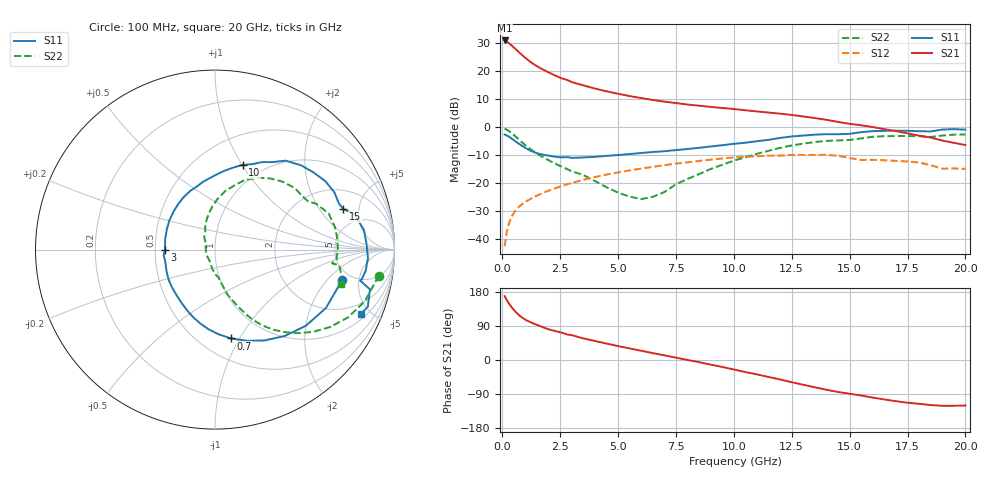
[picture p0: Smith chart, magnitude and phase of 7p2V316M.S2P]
! Infineon Technologies  Discrete & RF Semiconductors
! bfp620
! VCE =  2.3 V,  IC =  16 mA
! Common Emitter S-Parameters:  Sep 2002
# GHz  S  MA  R  50
!  f  S11  S21  S12  S22
! GHz  MAG  ANG  MAG  ANG  MAG  ANG  MAG  ANG
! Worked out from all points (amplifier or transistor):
!   59 points, 100 MHz to 20 GHz, reference 50 ohm
!   highest |S21| = 30.8 dB at 100 MHz (marker M1)
!   |S21| within 3 dB of that: start of sweep to 564.6 MHz
!   unconditionally stable (mu >= 1): 3.515 GHz to 10.17 GHz; 17.14 GHz to end of sweep
!   at 1 GHz: K = 0.65, MSG = 25.7 dB, |S12| = -26.8 dB
!   at 5.5 GHz: K = 1.05, MAG = 12.0 dB, |S12| = -15.6 dB
!   at 20 GHz: K = 1.27, MAG = 1.1 dB, |S12| = -15.0 dB
!   S11 on the Smith chart (normalised r, x): 100 MHz: 4.12, -2.98; 700 MHz: 0.70, -0.92; 3 GHz: 0.56, +0.00; 10 GHz: 0.80, +1.01; 15 GHz: 3.30, +3.40; 20 GHz: 1.29, -4.41
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0.1  0.7285 -13.5  34.74 168.6  0.0074 58.7  0.9239 -9.0
0.2  0.6985 -27.8  32.88 157.3  0.0138 66.3  0.8837 -18.9
0.3  0.6605 -40.0  30.71 147.8  0.0196 65.6  0.8318 -27.0
0.4  0.6185 -51.1  28.38 139.5  0.0246 63.5  0.7733 -33.9
0.5  0.5769 -61.3  26.05 132.1  0.0291 61.3  0.7132 -40.0
0.7  0.5034 -79.6  21.81 119.6  0.0367 57.7  0.601 -49.9
0.8  0.4723 -87.6  19.99 114.5  0.0399 56.3  0.552 -53.9
1  0.4198 -101.3  16.94 106.2  0.0458 54.5  0.4692 -59.9
1.2  0.3786 -112.8  14.58 100.1  0.0511 53.3  0.4046 -64.0
1.4  0.3484 -122.9  12.77 95.0  0.0564 52.4  0.3542 -67.1
2  0.3059 -148.4  9.363 81.1  0.0724 49.9  0.2532 -74.9
2.4  0.2878 -162.3  7.809 74.7  0.083 47.9  0.2088 -77.7
3  0.2787 179.9  6.268 65.6  0.0993 44.2  0.1608 -81.9
3.5  0.2837 168.2  5.489 57.0  0.1132 40.6  0.1379 -88.7
5  0.3131 137.5  3.88 36.7  0.1535 28.7  0.0668 -118.6
7  0.3662 105.8  2.812 12.4  0.2061 11.3  0.0684 141.8
10  0.4968 71.9  2.077 -25.0  0.2841 -20.0  0.2481 92.6
10.5  0.5195 66.4  1.972 -31.9  0.2917 -26.4  0.2867 86.5
13.5  0.7237 31.7  1.43 -72.0  0.3153 -61.4  0.5337 45.2
15  0.7488 17.6  1.129 -89.0  0.2774 -82.1  0.583 27.6
17  0.8534 -3.2  0.838 -108.7  0.2466 -93.0  0.6844 5.1
20  0.8895 -23.7  0.472 -120.1  0.1773 -103.3  0.7286 -15.4
